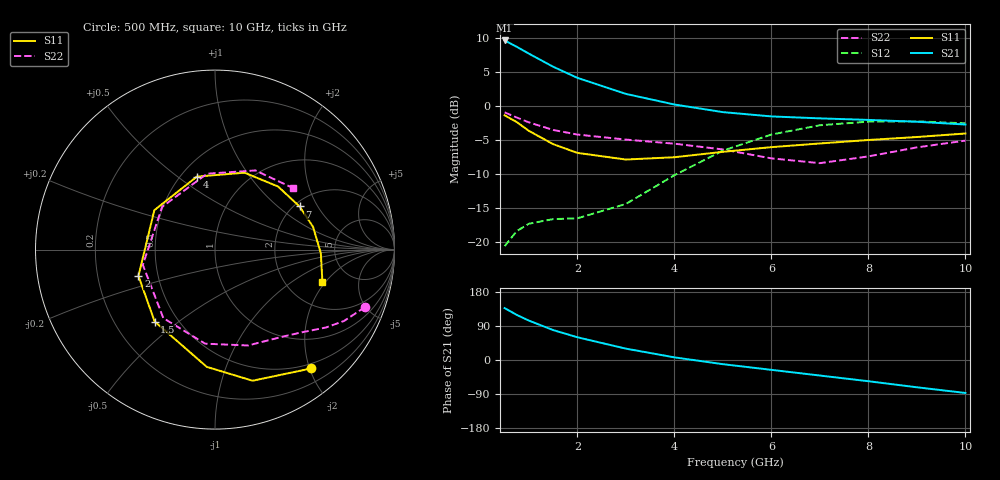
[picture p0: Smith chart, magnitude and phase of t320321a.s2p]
!AT-32032
!S-PARAMETERS at Vce=1V  Ic=1mA.  LAST UPDATED 05-29-98
# ghz s ma r 50
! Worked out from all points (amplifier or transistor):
!   13 points, 500 MHz to 10 GHz, reference 50 ohm
!   highest |S21| = 9.6 dB at 500 MHz (marker M1)
!   |S21| within 3 dB of that: start of sweep to 1.277 GHz
!   unconditionally stable (mu >= 1): 2.005 GHz to 3.553 GHz; 9.351 GHz to end of sweep
!   at 1 GHz: K = 0.51, MSG = 12.5 dB, |S12| = -17.3 dB
!   at 4 GHz: K = 0.93, MSG = 5.2 dB, |S12| = -10.2 dB
!   at 10 GHz: K = 1.00, MAG = -0.5 dB, |S12| = -2.6 dB
!   lowest NFmin = 1.10 dB at 900 MHz
!   S11 on the Smith chart (normalised r, x): 500 MHz: 0.42, -2.03; 1.5 GHz: 0.37, -0.41; 2 GHz: 0.39, -0.14; 4 GHz: 0.60, +0.59; 7 GHz: 2.14, +1.42; 10 GHz: 3.13, -1.88
0.5  0.852 -51.0  3.024 137.0  0.093 59.0  0.895 -21.0
0.75  0.76 -74.0  2.717 119.0  0.12 48.0  0.821 -29.0
1  0.655 -94.0  2.42 104.0  0.136 40.0  0.756 -35.0
1.5  0.523 -130.0  1.939 79.0  0.147 32.0  0.665 -44.0
2  0.451 -161.0  1.606 60.0  0.149 31.0  0.615 -52.0
3  0.403 147.0  1.224 30.0  0.19 43.0  0.565 -71.0
4  0.419 104.0  1.023 7.0  0.309 42.0  0.527 -96.0
5  0.459 69.0  0.899 -11.0  0.469 26.0  0.478 -127.0
6  0.497 45.0  0.836 -26.0  0.615 5.0  0.411 -168.0
7  0.529 27.0  0.809 -41.0  0.72 -18.0  0.379 141.0
8  0.561 13.0  0.788 -56.0  0.765 -40.0  0.425 96.0
9  0.59 -2.0  0.764 -72.0  0.769 -60.0  0.495 63.0
10  0.626 -17.0  0.729 -87.0  0.744 -79.0  0.555 38.0
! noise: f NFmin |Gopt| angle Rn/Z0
0.9  1.1  0.48  63  0.29
1.8  1.3  0.51  129  0.136
2  1.4  0.52  143  0.104
2.5  1.6  0.54  177  0.058
3  1.8  0.57  -153  0.098
3.5  2  0.61  -125  0.254
4  2.2  0.65  -102  0.52
